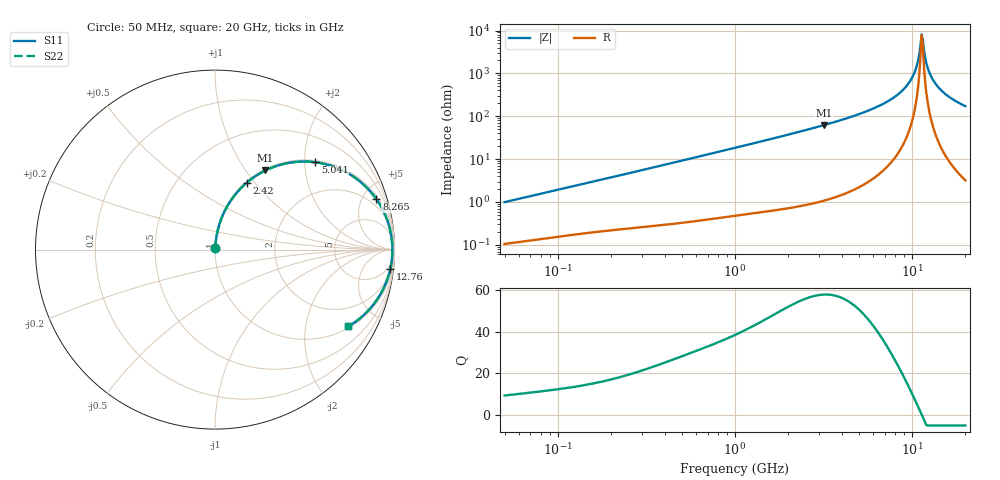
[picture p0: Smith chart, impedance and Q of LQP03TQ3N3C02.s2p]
!Murata Part Number: LQP03TQ3N3C02
!These Parameters are Measured in Series Mode Connection
!  o--[Z]--o
!Port1  Port2
!  o-------o
!Freq. Start=50[MHz] Stop=20[GHz], 401[Steps]
# Hz S RI R 50
!Freq.(Hz) S11(Real) S11(Imag) S21(Real) S21(Imag) S12(Real) S12(Imag) S22(Real) S22(Imag)
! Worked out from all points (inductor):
!   401 points, 50 MHz to 20 GHz, reference 50 ohm
!   read as one part in series: L = 3.11 nH near 51.52 MHz
!   highest Q = 57.9 at 3.169 GHz (marker M1), where L = 3.11 nH
!   self-resonance near 11.32 GHz
!   S11 on the Smith chart (normalised r, x): 50 MHz: 1.00, +0.02; 2.42 GHz: 1.02, +0.91; 5.041 GHz: 1.04, +2.26; 8.265 GHz: 1.26, +6.31; 12.76 GHz: 3, -17; 20 GHz: 1.06, -3.43
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5e7  0.00115 0.00986  0.9989 -0.00986  0.9989 -0.00986  0.00115 0.00986
1.364002e8  0.00249 0.0258  0.9975 -0.0258  0.9975 -0.0258  0.00249 0.0258
3.721004e8  0.00749 0.068  0.9925 -0.068  0.9925 -0.068  0.00749 0.068
1e9  0.0368 0.1757  0.9632 -0.1757  0.9632 -0.1757  0.0368 0.1757
2.419936e9  0.1775 0.3732  0.8225 -0.3732  0.8225 -0.3732  0.1775 0.3732
2.728004e9  0.2183 0.4044  0.7817 -0.4044  0.7817 -0.4044  0.2183 0.4044
3.168813e9  0.2807 0.4408  0.7193 -0.4408  0.7193 -0.4408  0.2807 0.4408
5.041459e9  0.5598 0.4866  0.4402 -0.4866  0.4402 -0.4866  0.5598 0.4866
7.442007e9  0.8383 0.3525  0.1617 -0.3525  0.1617 -0.3525  0.8383 0.3525
8.264682e9  0.8993 0.281  0.1007 -0.281  0.1007 -0.281  0.8993 0.281
9.316812e9  0.9522 0.1837  0.0478 -0.1837  0.0478 -0.1837  0.9522 0.1837
1.004137e10  0.974 0.1166  0.026 -0.1166  0.026 -0.1166  0.974 0.1166
1.050288e10  0.9824 0.0747  0.0176 -0.0747  0.0176 -0.0747  0.9824 0.0747
1.115139e10  0.988 0.0179  0.012 -0.0179  0.012 -0.0179  0.988 0.0179
1.131968e10  0.9883 0.00359  0.0117 -0.00359  0.0117 -0.00359  0.9883 0.00359
1.149051e10  0.9882 -0.0107  0.0118 0.0107  0.0118 0.0107  0.9882 -0.0107
1.166392e10  0.9878 -0.025  0.0122 0.025  0.0122 0.025  0.9878 -0.025
1.220001e10  0.9839 -0.0677  0.0161 0.0677  0.0161 0.0677  0.9839 -0.0677
1.276073e10  0.9763 -0.1098  0.0237 0.1098  0.0237 0.1098  0.9763 -0.1098
1.375312e10  0.9558 -0.1776  0.0442 0.1776  0.0442 0.1776  0.9558 -0.1776
1.504638e10  0.9193 -0.253  0.0807 0.253  0.0807 0.253  0.9193 -0.253
2e10  0.7424 -0.4281  0.2576 0.4281  0.2576 0.4281  0.7424 -0.4281
